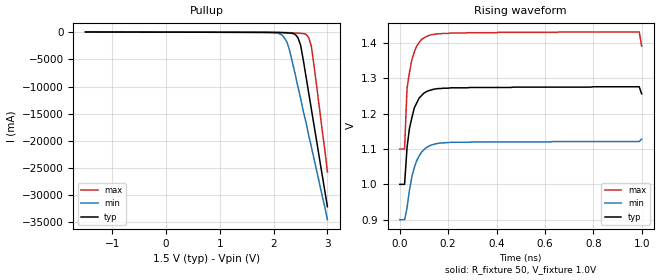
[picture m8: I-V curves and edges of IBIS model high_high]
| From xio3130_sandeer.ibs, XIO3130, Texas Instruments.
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[Model] high_high
Model_type Open_source
Polarity Non-Inverting
Cref = 2.0pF
Rref = 50
Vref = 1.0V
Vmeas =1.0V
|   typ   min   max
C_comp   1.603pF   1.594pF   1.637pF
[Temperature Range]   25   125   -40
[Voltage Range] 1.50V 1.35V 1.65V
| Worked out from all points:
|   slope of the pullup table from 0 to 0.225 V, typ, clamps not added: 45.9 ohm
|   rising waveform, R_fixture 50, V_fixture 1.0V: 20-80 % time 31ps typ, 49.7ps min, 21.3ps max; typ from 1 V to 1.26 V
| (Process strength) nominal weak strong
[Pullup]
-1.5V     32.94mA    32.2mA     33.5mA
1.8V      -38.72mA   -49.27mA   -39.53mA
2.15V     -93.3mA    -494.3mA   -53.96mA
2.25V     -140.6mA   -1.883A    -78.67mA
2.3V      -170.8mA   -3.488A    -98.89mA
2.45V     -985.3mA   -9.998A    -185.6mA
2.5V      -2.318A    -12.1A     -221.3mA
2.6V      -8.049A    -16.5A     -382.6mA
2.65V     -11.05A    -18.9A     -953.2mA
2.7V      -14.06A    -21A       -2.52A
2.75V     -17.07A    -23.3A     -6.046A
3V        -32.12A    -34.5A     -25.7A
[Ramp]
| variable   typ   min   max
dV/dt_r 0.24618V/0.0415301ns  0.25194V/0.0445372ns  0.243V/0.0389342ns
dV/dt_f 0.23754V/0.0399045ns  0.23268V/0.0376058ns  0.2367V/0.0389008ns
R_load = 50
[Rising Waveform]
R_fixture = 50
V_fixture = 1.0V
V_fixture_min = 0.9V
V_fixture_max = 1.1V
0s        1V         900mV      1.1V
20ps      1V         900mV      1.1V
30ps      1.103V     933.4mV    1.271V
40ps      1.158V     982.9mV    1.316V
50ps      1.188V     1.021V     1.352V
80ps      1.244V     1.08V      1.401V
120ps     1.265V     1.108V     1.421V
210ps     1.273V     1.119V     1.428V
990ps     1.276V     1.121V     1.431V
1ns       1.256V     1.128V     1.391V
